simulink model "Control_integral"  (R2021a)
settings: Solver=ode45  StartTime=0.0  StopTime=0.02  MaxStep=1e-4  RelTol=1e-3  EnableMultiTasking=on
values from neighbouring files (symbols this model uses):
  Am = [-R1/L1 R1/L1; R1/L2 -(R1+R2)/L2]    [Clase_25_11_2021_Inte.m]
  Bm = [-1/L1;0]    [Clase_25_11_2021_Inte.m]
  R2 = 5    [Clase_25_11_2021_Inte.m]

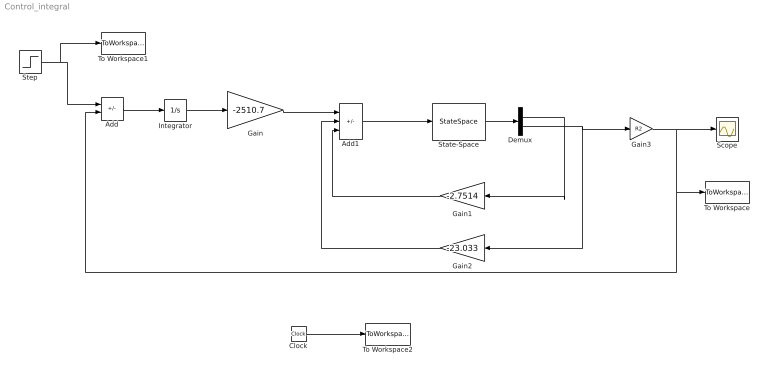
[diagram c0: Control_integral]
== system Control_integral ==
  Add : Sum  Inputs=-+
  Add1 : Sum  Inputs=---
  Clock : Clock
  Demux : Demux  Outputs=2
  Gain : Gain  Gain=-2510.7
  Gain1 : Gain  Gain=-2.7514
  Gain2 : Gain  Gain=-23.033
  Gain3 : Gain  Gain=R2
  Integrator : Integrator
  Scope : Scope
  State-Space : StateSpace  A=Am  B=Bm  C=[1 0;0 1]  D=[0;0]  InitialCondition=0
  Step : Step  Time=0.01  After=50  SampleTime=0
  To Workspace : ToWorkspace  VariableName=E  SampleTime=-1
  To Workspace1 : ToWorkspace  VariableName=in  SampleTime=-1
  To Workspace2 : ToWorkspace  VariableName=time  SampleTime=-1
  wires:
  Step/1 -> To Workspace1/1, Add/1
  Add/1 -> Integrator/1
  Integrator/1 -> Gain/1
  Gain/1 -> Add1/1
  Add1/1 -> State-Space/1
  State-Space/1 -> Demux/1
  Demux/1 -> Gain1/1
  Demux/2 -> Gain3/1, Gain2/1
  Gain1/1 -> Add1/3
  Gain2/1 -> Add1/2
  Gain3/1 -> Add/2, To Workspace/1, Scope/1
  Clock/1 -> To Workspace2/1
